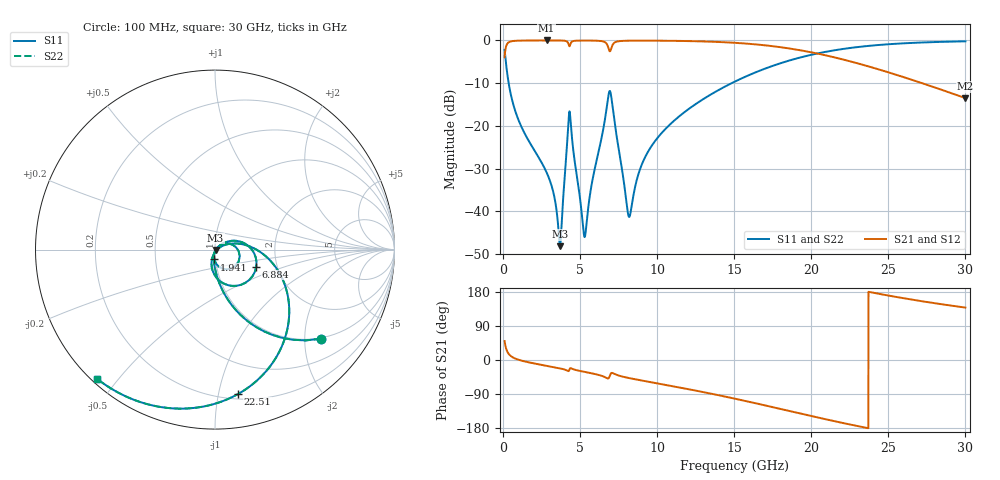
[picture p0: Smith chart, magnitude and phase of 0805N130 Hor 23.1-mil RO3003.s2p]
# GHz S MA R 50
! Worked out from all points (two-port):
!   3201 points, 100 MHz to 30 GHz, reference 50 ohm
!   highest |S21| = -0.02 dB at 2.819 GHz (marker M1); lowest = -13.5 dB at 30 GHz (marker M2)
!   |S21| within 3 dB of the highest: 121.3 MHz to 20.32 GHz (20.2 GHz wide, 198 % of centre)
!   lowest |S11| = -48.1 dB at 3.697 GHz (marker M3), VSWR 1.01, Z = 50.3 - j0.19 ohm
!   |S11| at or under -10 dB: 362.9 MHz to 14.84 GHz (14.47 GHz wide, 190 % of centre)
!   |S22| runs from -48.1 to -0.2 dB; largest |S21 - S12| = 0
!   S11 on the Smith chart (normalised r, x): 100 MHz: 0.98, -2.40; 1.941 GHz: 0.98, -0.11; 6.884 GHz: 1.56, -0.32; 22.51 GHz: 0.24, -1.15; 30 GHz: 0.02, -0.44
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0.1  0.7716 -40.1  0.6357 49.9  0.6357 49.9  0.7716 -40.1
0.5017812  0.2337 -79.3  0.9716 10.5  0.9716 10.5  0.2337 -79.3
1.940719  0.05509 -96.9  0.9969 -8.5  0.9969 -8.5  0.05509 -96.9
2.819031  0.02873 -101.3  0.9975 -15.2  0.9975 -15.2  0.02873 -101.3
3.267531  0.01658 -100.1  0.9973 -18.6  0.9973 -18.6  0.01658 -100.1
3.697344  0.003926 -28.7  0.996 -22.1  0.996 -22.1  0.003926 -28.7
3.818812  0.008302 29.0  0.9947 -23.2  0.9947 -23.2  0.008302 29.0
4.192563  0.0807 24.7  0.9497 -28.7  0.9497 -28.7  0.0807 24.7
4.314031  0.1477 -33.3  0.8536 -24.4  0.8536 -24.4  0.1477 -33.3
5.089563  0.01006 -87.8  0.9945 -29.7  0.9945 -29.7  0.01006 -87.8
5.360531  0.005765 -2.4  0.9948 -31.9  0.9948 -31.9  0.005765 -2.4
6.60325  0.1168 25.1  0.9542 -45.2  0.9542 -45.2  0.1168 25.1
6.883563  0.2488 -22.5  0.7669 -46.2  0.7669 -46.2  0.2488 -22.5
7.247969  0.1063 -99.0  0.9452 -37.1  0.9452 -37.1  0.1063 -99.0
8.173  0.008627 -43.8  0.9911 -47.6  0.9911 -47.6  0.008627 -43.8
8.967219  0.03407 25.5  0.9928 -53.9  0.9928 -53.9  0.03407 25.5
10.06978  0.07423 23.5  0.9912 -62.1  0.9912 -62.1  0.07423 23.5
15.05  0.3302 -13.4  0.9362 -102.1  0.9362 -102.1  0.3302 -13.4
20.03956  0.6805 -59.0  0.7228 -148.2  0.7228 -148.2  0.6805 -59.0
22.50631  0.8143 -80.8  0.5698 -170.2  0.5698 -170.2  0.8143 -80.8
25.01978  0.9013 -100.7  0.4219 169.9  0.4219 169.9  0.9013 -100.7
30  0.9744 -132.2  0.2113 138.3  0.2113 138.3  0.9744 -132.2
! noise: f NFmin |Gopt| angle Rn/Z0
0.1  0.00066  0.9069  0.936  0.001555
3.417  0.007314  0.7398  20.46  0.005457
6.743  0.06064  0.9331  39.64  0.1785
10.06  0.01757  0.707  57.54  0.009139
13.39  0.02152  0.6968  73.89  0.009015
16.7  0.02736  0.7128  88.85  0.009838
20.03  0.03517  0.7402  102.7  0.01094
23.35  0.04592  0.7754  115.8  0.01228
26.67  0.06164  0.8162  128.5  0.01384
30  0.08614  0.8593  140.9  0.01535
